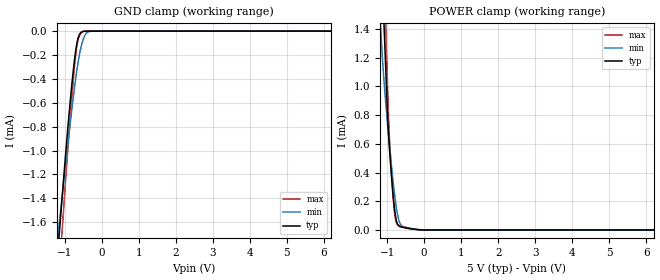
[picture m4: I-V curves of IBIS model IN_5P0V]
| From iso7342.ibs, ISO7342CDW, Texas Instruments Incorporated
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|   Model IN_5P0V
[Model]   IN_5P0V
Model_type   Input
Vinl = .8
Vinh = 2
|   typ   min   max
|   (nom PVT)   (slow PVT)   (fast PVT)
C_comp   0.354p   0.325p   0.383p
| Where   nom PVT is  Nominal Process, 5.0V, 27C
|   Fast PVT is Strong Process, 5.5V, -40C
|   Slow PVT is Weak Process, 4.5V, 150C
[Voltage Range]   5   4.5   5.5
[Temperature Range]   27   150   -40
[Power Clamp Reference]   5   4.5   5.5
[GND Clamp Reference]   0   0   0
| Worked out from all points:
|   GND clamp passes 1 mA (typ) near -0.96 V on its own axis
|   POWER clamp passes 1 mA (typ) near -1.02 V on its own axis
[GND Clamp]
|   Voltage   I(typ)   I(min)   I(max)
-5V       -17.49mA   -13.39mA   -21.79mA
-1.265V   -2.166mA   -1.968mA   -2.56mA
-1.13V    -1.641mA   -1.569mA   -1.954mA
-1.115V   -1.583mA   -1.526mA   -1.887mA
-1.055V   -1.349mA   -1.352mA   -1.617mA
-875mV    -679.6uA   -844.2uA   -834.7uA
-740mV    -259.5uA   -491.7uA   -320.4uA
-650mV    -75.81uA   -288.9uA   -93.96uA
-515mV    -4.2uA     -86.9uA    -5.717uA
-410mV    -367.7nA   -16.42uA   -267.5nA
-290mV    -148.8nA   -1.483uA   -81.78nA
10V       0A         0A         0A
[POWER Clamp]
|   Voltage   I(typ)   I(min)   I(max)
-5V       33.7mA     25.28mA    41.1mA
-1.265V   2.636mA    1.846mA    3.37mA
-1.13V    1.74mA     1.206mA    2.217mA
-1.085V   1.441mA    1.042mA    1.833mA
-1.04V    1.143mA    894.1uA    1.449mA
-1.025V   1.043mA    847.5uA    1.321mA
-980mV    744.9uA    713.8uA    937.1uA
-950mV    621.2uA    628.7uA    718.6uA
-845mV    264uA      354.7uA    250.1uA
-770mV    92.28uA    191.7uA    69.37uA
-650mV    23.46uA    45.43uA    29.88uA
10V       0A         0A         0A
